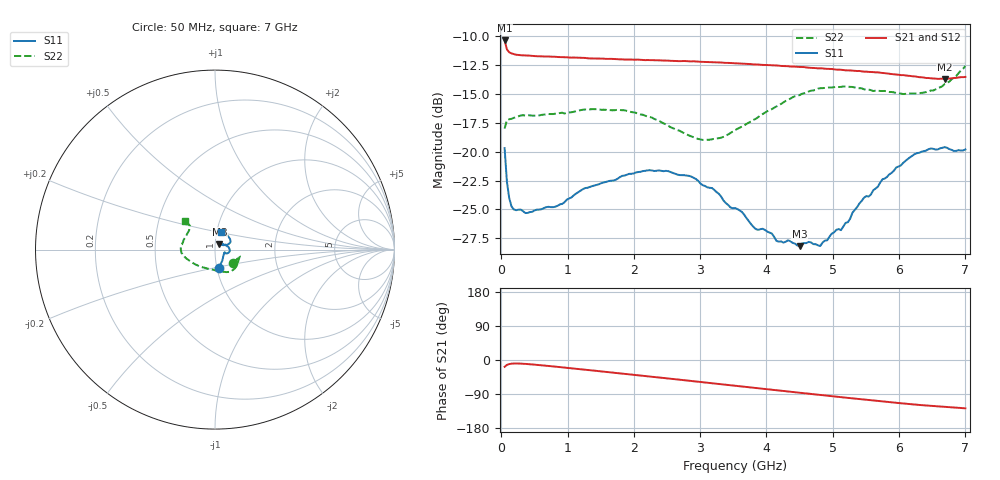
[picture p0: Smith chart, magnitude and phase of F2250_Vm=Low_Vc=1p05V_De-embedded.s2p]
! Integrated Device Technology
! Corporate Headquarters
! 6024 Silver Creek Valley Road
! San Jose, CA 95138  USA
! Phone:  1-408-284-8200
! Toll Free:  1-800-223-1366
! Webpage:  http://www.idt.com/
! Timing and RF Division
! 515 Groton Road, Suite 102
! Westford, MA 01886-6024
! Device:  F2250
! Description: Voltage Variable RF Attenuator
! Frequency:  50.0 -  6000.00 MHz
! Package:  3x3 mm Thin QFN Plastic Package: 16 pin
! Ports:  2 RF, 3 DC
!  Pin  1  = GND
!  Pin  2  = NC
!  Pin  3  = RF1  = Port 1
!  Pin  4  = NC
!  Pin  5  = GND
!  Pin  6  = GND
!  Pin  7  = GND
!  Pin  8  = GND
!  Pin  9  = NC
!  Pin 10  = RF2  = Port 2
!  Pin 11  = NC
!  Pin 12  = GND
!  Pin 13  = GND
!  Pin 14  = VCNTRL
!  Pin 15  = VDD
!  Pin 16  = VMODE
! Vcntrl:  1.050 Volts
! Vmode:  +0.000 Volts
! Vdd:  +3.30  Volts
! Current:  1.188 mA
! Data:  The device was measured on a the F2250 evaluation board which has
!  individual transmission lines to the RF pins.  Data was collected
!  using a calibrated network analyzer.  The evaluation board was
!  de-embedded using a TRL calibration technique.
!  The reference plane is the edge of the package pin.
! Misc:  SN 10
!  Action Tracker AT0258
! Date Measured:  2014-11-26
! Date:  2015-10-15  MJV
! Note:
!  Integrated Device Technology supplies this data as a sample of measured
!  data at the package pin for this product.  Your particular data for this
!  product may vary.
!  Data was taken at 25 degrees C.
!  Integrated Device Technology reserves the right to change this data at anytime.
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# GHz S dB R 50
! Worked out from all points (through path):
!   201 points, 50 MHz to 7 GHz, reference 50 ohm
!   highest |S21| = -10.40 dB at 50 MHz (marker M1); lowest = -13.7 dB at 6.687 GHz (marker M2)
!   group delay of S21, straight-line fit = 50.5 ps
!   lowest |S11| = -28.2 dB at 4.498 GHz (marker M3), VSWR 1.08, Z = 52.4 + j3.17 ohm
!   |S11| at or under -10 dB: start of sweep to end of sweep
!   |S22| runs from -19.0 to -12.6 dB; largest |S21 - S12| = 0.00057
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0.05  -19.70 -78.5  -10.40 -18.0  -10.41 -18.0  -18.02 -36.0
0.08475  -22.61 -56.7  -11.17 -12.9  -11.19 -12.9  -17.28 -20.1
0.1195  -24.02 -45.5  -11.42 -10.7  -11.42 -10.7  -17.21 -15.4
0.189  -25.00 -31.6  -11.58 -9.3  -11.59 -9.3  -17.08 -13.6
0.3975  -25.30 -18.9  -11.71 -10.7  -11.71 -10.7  -16.86 -16.1
0.8145  -24.77 -16.8  -11.81 -17.5  -11.80 -17.5  -16.72 -29.0
1.2315  -23.25 -17.9  -11.91 -25.0  -11.90 -25.0  -16.38 -40.4
1.857  -22.08 -11.3  -12.05 -36.4  -12.04 -36.4  -16.43 -53.8
2.37825  -21.63 -2.6  -12.11 -46.1  -12.11 -46.1  -17.32 -66.7
2.86475  -22.16 9.1  -12.21 -55.3  -12.19 -55.3  -18.68 -87.8
3.0385  -22.90 13.6  -12.25 -58.6  -12.24 -58.6  -18.99 -98.1
3.525  -24.88 28.0  -12.38 -67.9  -12.37 -67.9  -18.15 -128.9
3.83775  -26.70 39.9  -12.47 -73.8  -12.46 -73.8  -17.17 -144.5
4.498  -28.17 50.8  -12.68 -86.4  -12.67 -86.4  -15.12 -167.9
4.7065  -28.00 50.0  -12.77 -90.3  -12.76 -90.3  -14.72 -172.4
4.81075  -28.16 44.8  -12.80 -92.2  -12.79 -92.3  -14.52 -174.3
5.1235  -26.79 35.2  -12.93 -98.1  -12.93 -98.1  -14.41 178.5
5.471  -23.98 25.8  -13.10 -104.3  -13.08 -104.4  -14.62 170.9
5.85325  -21.96 21.9  -13.27 -111.2  -13.28 -111.2  -14.85 160.8
6.2355  -20.21 27.2  -13.50 -117.6  -13.50 -117.6  -14.99 148.2
6.68725  -19.62 45.2  -13.73 -123.3  -13.71 -123.4  -14.16 136.3
7  -19.82 69.7  -13.55 -127.6  -13.54 -127.7  -12.60 136.3
